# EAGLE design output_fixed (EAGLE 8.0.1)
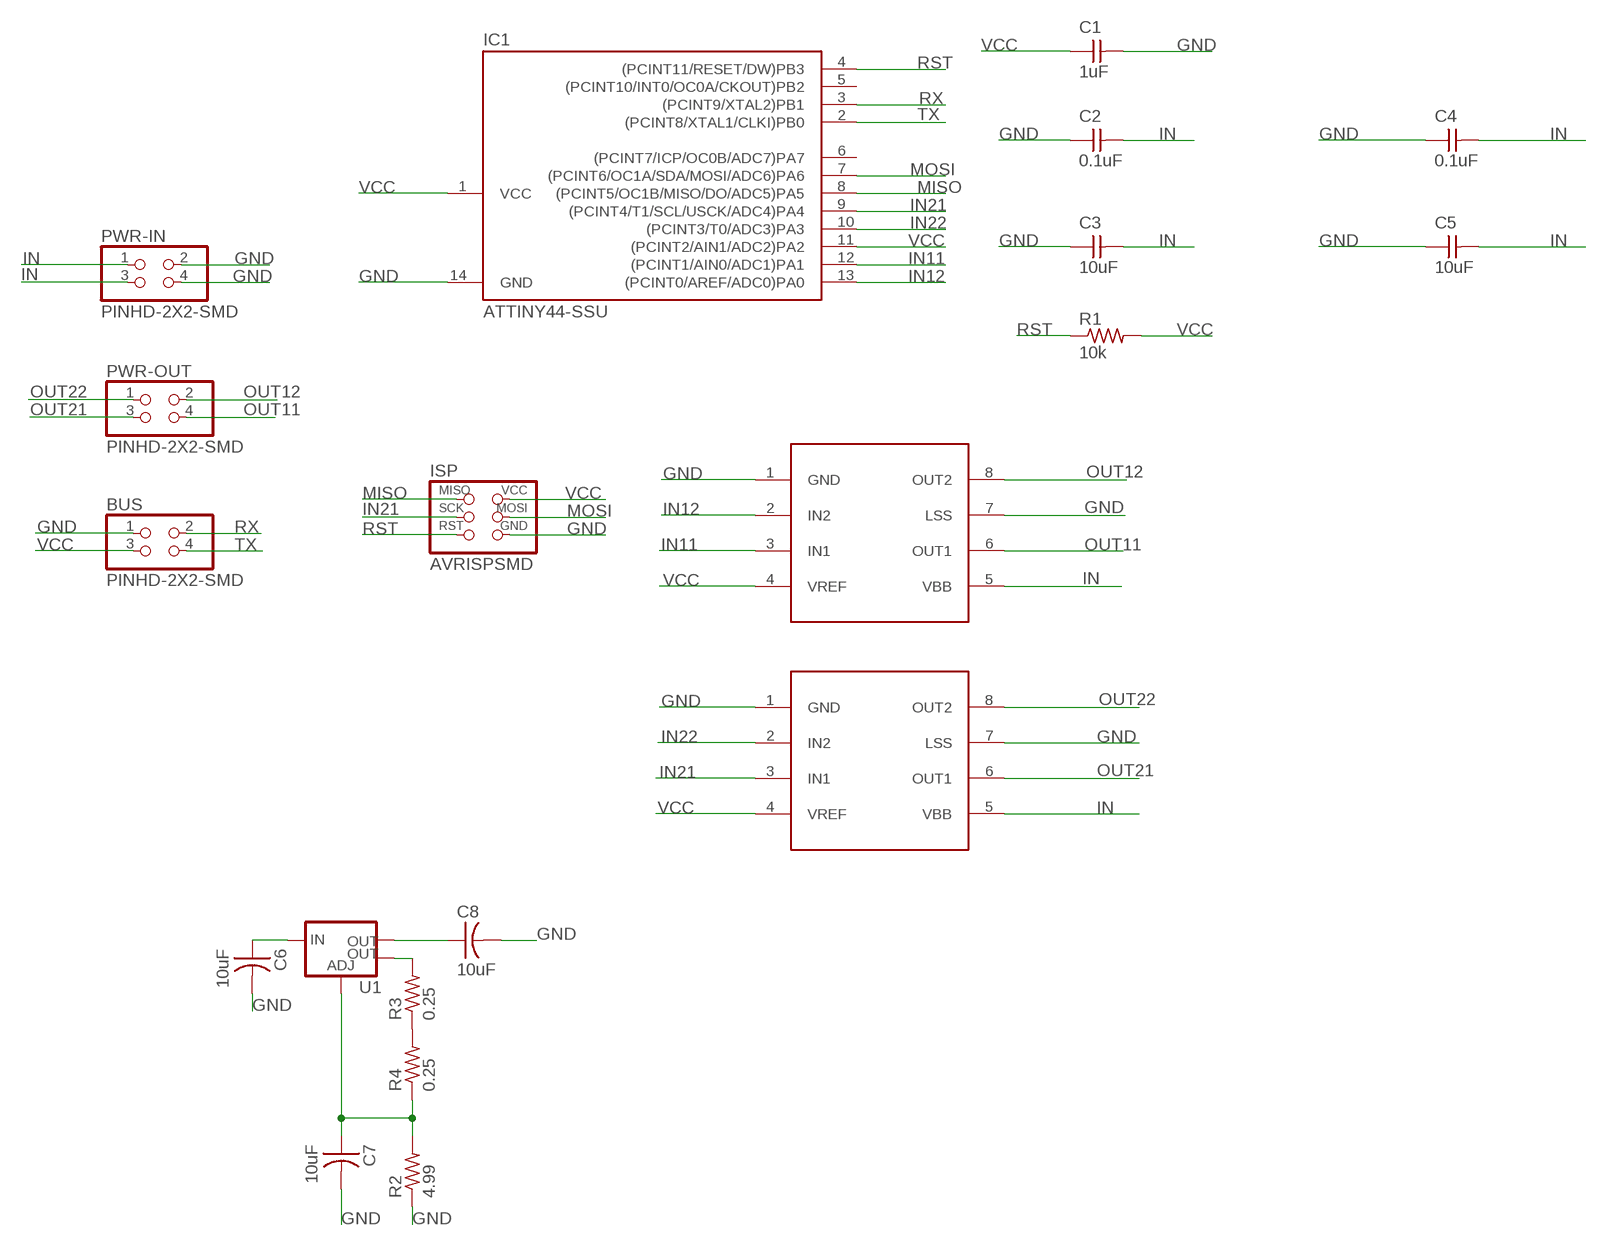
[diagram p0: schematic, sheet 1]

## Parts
BUS  PINHD-2X2-SMD  [2X02SMD]
C1  1uF  CAP-UNPOLARIZEDFAB  [C1206FAB]
C2  0.1uF  CAP-UNPOLARIZEDFAB  [C1206FAB]
C3  10uF  CAP-UNPOLARIZEDFAB  [C1206FAB]
C4  0.1uF  CAP-UNPOLARIZEDFAB  [C1206FAB]
C5  10uF  CAP-UNPOLARIZEDFAB  [C1206FAB]
C6  10uF  CAP-US1206FAB  [C1206FAB]
C7  10uF  CAP-US1206FAB  [C1206FAB]
C8  10uF  CAP-US1206FAB  [C1206FAB]
IC1  ATTINY44-SSU  [SOIC14]
ISP  AVRISPSMD  [2X03SMD]
PWR-IN  PINHD-2X2-SMD  [2X02SMD]
PWR-OUT  PINHD-2X2-SMD  [2X02SMD]
R1  10k  RES-US1206FAB  [R1206FAB]
R2  4.99  RES-US1206FAB  [R1206FAB]
R3  0.25  RES-US1206FAB  [R1206FAB]
R4  0.25  RES-US1206FAB  [R1206FAB]
U1  V_REG_LM1117SOT223  [SOT223]
U$5  A4953-H-BRIDGE-MOTOR-DRIVER  [SOIC8]
U$6  A4953-H-BRIDGE-MOTOR-DRIVER  [SOIC8]

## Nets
GND: BUS.1 C1.2 C2.1 C3.1 C4.1 C5.1 C6.2 C7.2 C8.2 IC1.14(GND) ISP.6(GND) PWR-IN.2 PWR-IN.4 R2.1 U$5.1(GND) U$5.7(LSS) U$6.1(GND) U$6.7(LSS)
IN: C2.2 C3.2 C4.2 C5.2 PWR-IN.1 PWR-IN.3 U$5.5(VBB) U$6.5(VBB)
IN11: IC1.12((PCINT1/AIN0/ADC1)PA1) U$5.3(IN1)
IN12: IC1.13((PCINT0/AREF/ADC0)PA0) U$5.2(IN2)
IN21: IC1.9((PCINT4/T1/SCL/USCK/ADC4)PA4) ISP.3(SCK) U$6.3(IN1)
IN22: IC1.10((PCINT3/T0/ADC3)PA3) U$6.2(IN2)
MISO: IC1.8((PCINT5/OC1B/MISO/DO/ADC5)PA5) ISP.1(MISO)
MOSI: IC1.7((PCINT6/OC1A/SDA/MOSI/ADC6)PA6) ISP.4(MOSI)
N$1: C6.1 U1.3(IN)
N$2: C7.1 R2.2 R4.1 U1.1(ADJ)
N$3: C8.1 U1.2(OUT)
N$4: R3.2 U1.4(OUT)
N$5: R3.1 R4.2
OUT11: PWR-OUT.4 U$5.6(OUT1)
OUT12: PWR-OUT.2 U$5.8(OUT2)
OUT21: PWR-OUT.3 U$6.6(OUT1)
OUT22: PWR-OUT.1 U$6.8(OUT2)
RST: IC1.4((PCINT11/RESET/DW)PB3) ISP.5(RST) R1.1
RX: BUS.2 IC1.3((PCINT9/XTAL2)PB1)
TX: BUS.4 IC1.2((PCINT8/XTAL1/CLKI)PB0)
VCC: BUS.3 C1.1 IC1.1(VCC) IC1.11((PCINT2/AIN1/ADC2)PA2) ISP.2(VCC) R1.2 U$5.4(VREF) U$6.4(VREF)
Unconnected: IC1.5((PCINT10/INT0/OC0A/CKOUT)PB2) IC1.6((PCINT7/ICP/OC0B/ADC7)PA7)

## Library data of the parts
BUS PWR-IN PWR-OUT = fab:PINHD-2X2-SMD
C1-C5 = fab:CAP-UNPOLARIZED
C6-C8 = fab:CAP-US
IC1 = fab:ATTINY44
ISP = fab:AVRISP
R1-R4 = fab:RES-US: Resistor (US Symbol)
U1 = fab:V_REG_LM1117: Voltage Regulator LM1117 Standard adjustable voltage regulator but in SMD form. Spark Fun Electronics SKU : COM-00595; PROD_ID: VREG-08170
U$5 U$6 = fab:A4953-H-BRIDGE-MOTOR-DRIVER

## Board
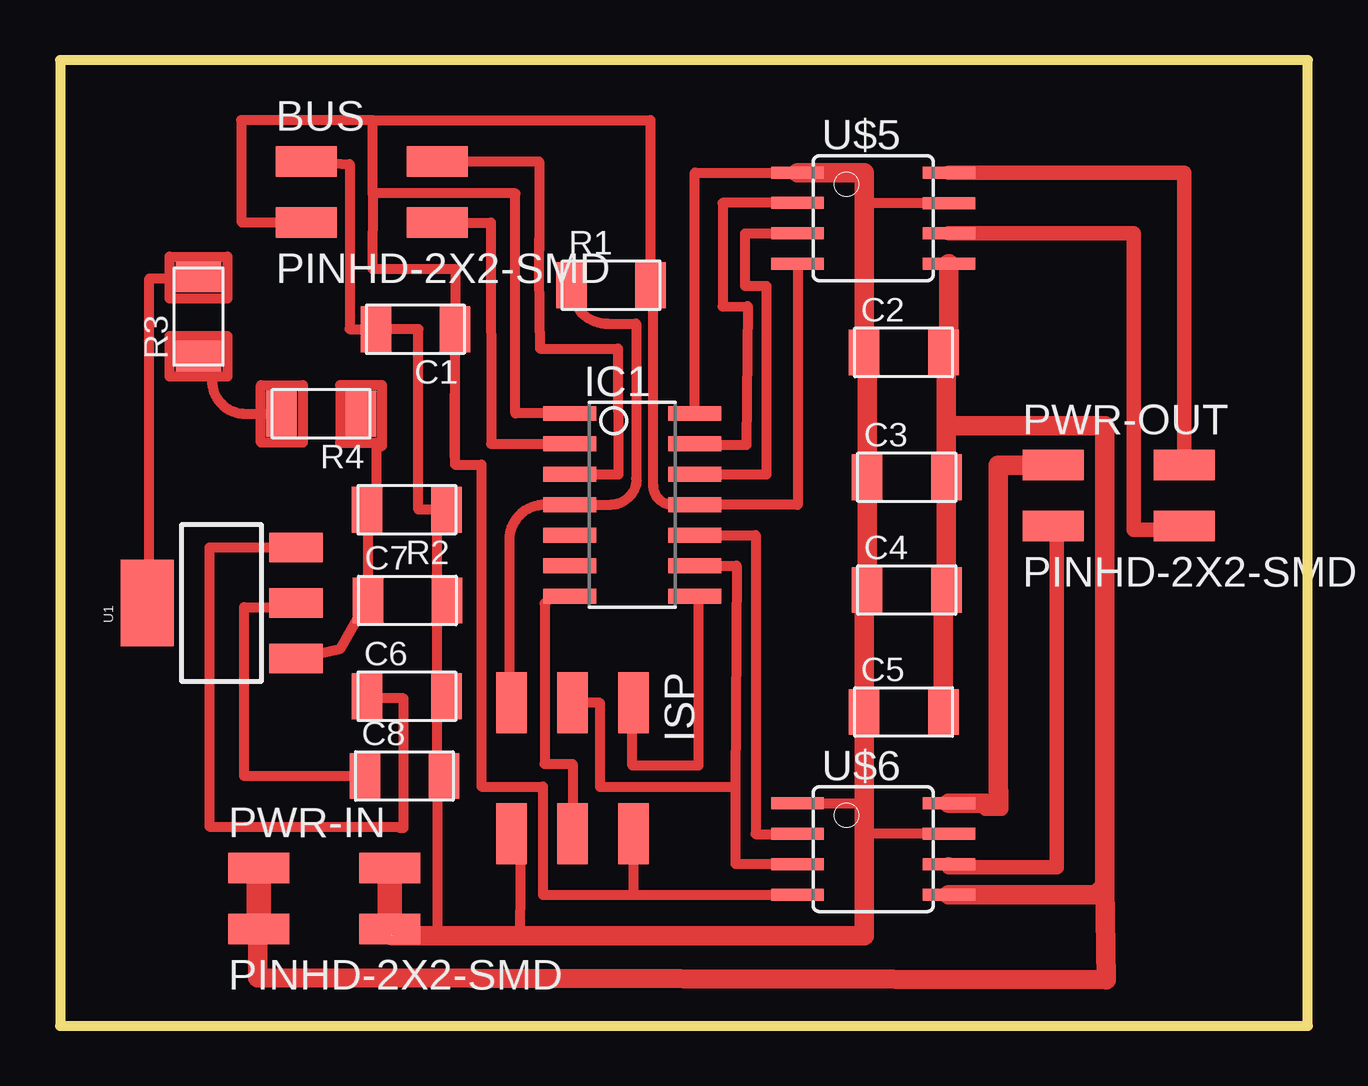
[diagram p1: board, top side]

Size 51.99 x 40.25 mm. Coordinates in mm from the lower left corner, seen from the top.
Outline: 0,0 51.99,0 51.99,40.25 0,40.25 0,0
Copper layers (1*16): Top 0.035mm / dielectric 1.5mm / Bottom 0.035mm
Design rules "default": minimum track width 10mil, minimum drill 24mil, track to track 8mil, track to pad 8mil, pad to pad 8mil, via to via 8mil, smd to smd 8mil, copper to edge 40mil, drill to drill 8mil, minimum pad ring 10mil, minimum via ring 8mil, stop-mask expansion 4mil, vias tented up to drill 0mil, thermal gap 10mil

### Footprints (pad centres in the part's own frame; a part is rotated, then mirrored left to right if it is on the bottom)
2X02SMD = smd 2.54 x 1.27: 1 -2.54,1.27; 2 2.92,1.27; 3 -2.54,-1.27; 4 2.92,-1.27
C1206FAB = smd 1.27 x 1.905: 1 -1.651,0; 2 1.651,0
SOIC14 = smd 0.61 x 2.21: 1 -3.81,-2.603; 2 -2.54,-2.603; 3 -1.27,-2.603; 4 0,-2.603; 5 1.27,-2.603; 6 2.54,-2.603; 7 3.81,-2.603; 8 3.81,2.603; 9 2.54,2.603; 10 1.27,2.603; 11 0,2.603; 12 -1.27,2.603; 13 -2.54,2.603; 14 -3.81,2.603
2X03SMD = smd 2.54 x 1.27: 1 -2.54,2.54; 2 2.92,2.54; 3 -2.54,0; 4 2.92,0; 5 -2.54,-2.54; 6 2.92,-2.54
R1206FAB = smd 1.27 x 1.905: 1 -1.651,0; 2 1.651,0
SOT223 = smd 1.219 x 2.235: 1 -2.311,-3.099; 2 0,-3.099; 3 2.311,-3.099 | smd 3.6 x 2.2: 4 0,3.099
SOIC8 = smd 0.5 x 2.2: 1 -1.905,-3.154; 2 -0.645,-3.154; 3 0.625,-3.154; 4 1.895,-3.154; 5 1.905,3.154; 6 0.635,3.154; 7 -0.635,3.154; 8 -1.905,3.154

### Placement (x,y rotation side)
BUS  12.8,34.75 0 top
C1  14.81,29.03 180 top
C2  35.15,28.07 0 top
C3  35.28,22.86 0 top
C4  35.28,18.16 0 top
C5  35.15,13.08 0 top
C6  14.45,13.74 0 top
C7  14.48,17.73 0 top
C8  14.35,10.41 0 top
IC1  23.85,21.72 270 top
ISP  21.36,10.92 270 top
PWR-IN  10.82,5.31 0 top
PWR-OUT  43.92,22.1 0 top
R1  22.96,30.86 0 top
R2  14.45,21.51 180 top
R3  5.77,29.56 90 top
R4  10.88,25.51 180 top
U1  6.73,17.62 90 top
U$5  33.88,33.66 270 top
U$6  33.88,7.37 270 top

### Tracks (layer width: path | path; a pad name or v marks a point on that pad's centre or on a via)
GND  (1 unrouted)
  Top 0.305: 15.72,21.51 R2.1 | C7.2 15.72,17.73 15.72,17.14 | C6.2 15.72,13.74 15.72,13.34 | C8.2 15.72,10.41 15.72,10.79
  Top 0.406: ISP.6 19.2,8.05 19.15,3.76 | U$6.7 33.5,8 | U$6.1 33.5,9.27 | U$5.7 33.5,34.29 | 33.5,25.53 33.63,25.65 | IC1.14 26.45,35.56 U$5.1 | BUS.1 12.06,35.92 12.06,29.03 C1.2 | C1.2 13.74,29.03 | C1.2 14.94,29.03 14.94,21.51 R2.1 | 15.72,21.51 15.72,17.14 15.72,13.34 15.72,10.79 15.72,3.76
  Top 0.813: 13.82,3.79 PWR-IN.2 | 13.84,3.76 15.72,3.76 19.15,3.76 33.5,3.76 33.5,8 33.5,9.27 C5.1 33.5,18.03 C4.1 C3.1 33.63,25.65 33.63,27.94 C2.1 33.5,34.29 33.5,35.56 U$5.1
  Top 1.016: PWR-IN.2 PWR-IN.4
IN
  Top 0.406: 36.8,18.16 C4.2 36.8,18.03 | C2.2 36.93,27.94 | PWR-IN.1 8.31,6.98 8.23,6.58
  Top 0.813: U$5.5 37.04,28.68 C2.2 | C5.2 36.8,18.03 | C4.2 C3.2 36.93,25.02 | 36.93,25.02 43.54,25.02 43.54,5.84 | 43.54,5.84 43.15,5.46 U$6.5 | 36.93,27.94 36.93,25.02 | 8.23,6.58 8.23,2.01 43.59,1.93 43.54,5.84
  Top 1.016: PWR-IN.1 PWR-IN.3
IN11
  Top 0.406: IC1.12 29.44,22.99 29.44,30.84 28.55,30.84 28.55,33.02 30.72,33.02 U$5.3
IN12
  Top 0.406: U$5.2 27.61,34.3 27.61,29.97 28.65,30 28.6,24.21 26.45,24.21 IC1.13
IN21
  Top 0.406: IC1.9 28.19,19.18 28.14,9.96 | 30.61,6.73 U$6.3 28.14,6.75 28.14,9.96 | 28.14,9.96 22.5,9.96 22.5,13.46 ISP.3
IN22
  Top 0.406: 30.59,8 U$6.2 30.73,8 28.98,8 28.98,20.45 IC1.10
MISO
  Top 0.406: IC1.8 26.59,17.91 26.59,10.85 23.85,10.85 23.85,13.46 ISP.1
MOSI
  Top 0.406: IC1.7 20.5,17.91 20.19,17.6 20.19,10.92 21.36,10.92 ISP.4 21.31,7.26
N$1
  Top 0.305: C6.1 12.8,13.55
  Top 0.406: U1.3 6.22,19.93 6.22,8.3 14.17,8.3 14.17,8.25 14.32,8.25 14.32,13.66 12.8,13.66 C6.1
N$2
  Top 0.305: 13.18,22.23 12.8,22.23 R2.2
  Top 0.406: 13.18,24.16 13.18,22.23 | U1.1 11.68,15.71 C7.1 12.83,21.51 R2.2 | 13.18,24.16 13.42,24.16 13.42,26.7 11.67,26.7 11.67,24.3 12.72,24.3 | 12.72,24.3 13.18,24.3 13.18,24.16 | 12.72,24.3 12.53,24.3 R4.1
N$3
  Top 0.305: 9.93,17.45 U1.2
  Top 0.406: C8.1 7.67,10.41 7.67,17.45 9.93,17.45
N$4
  Top 0.305: U1.4 3.72,17.27
  Top 0.406: 4.57,31.15 4.57,32.05 6.97,32.05 6.97,30.3 4.57,30.3 4.57,31.15 | 4.57,31.15 5.77,31.15 R3.2 | 4.57,31.15 3.72,31.15 3.72,17.27
N$5
  Top 0.305: R3.1 6.33,28.21
  Top 0.406: 6.33,28.21 6.33,27.05 | 6.33,27.05 4.57,27.05 4.57,28.76 6.97,28.76 6.97,27.05 6.33,27.05 | 6.33,27.05 6.33,26.89 arc90 7.72,25.5 8.37,25.5 | 8.37,25.5 R4.2 | R4.2 arc90 R4.2 | 8.37,25.5 8.37,26.7 10.12,26.7 10.12,24.3 8.37,24.3 8.37,25.5
OUT11
  Top 0.406: 46.84,20.68 PWR-OUT.4
  Top 0.61: U$5.6 44.73,33.02 44.73,20.68 46.84,20.68
OUT12
  Top 0.61: U$5.8 46.84,35.56 PWR-OUT.2
OUT21
  Top 0.61: PWR-OUT.3 41.53,20.83 41.53,6.6 37.04,6.6 U$6.6
OUT22
  Top 0.61: 39.09,9.78 39.22,9.78 39.22,9.04 38.58,9.04 38.58,9.27
  Top 0.813: U$6.8 38.58,9.27 | 39.09,9.78 39.09,23.37 PWR-OUT.1
RST
  Top 0.406: 21.25,21.67 IC1.4 | IC1.4 20.18,21.72 arc90 18.72,20.25 18.72,13.46 ISP.5 | IC1.4 22.93,21.72 arc90 24.02,22.8 24,22.8 24,29.26 22.82,29.26 22.82,29.26 arc-90 21.31,30.77 R1.1
RX
  Top 0.406: IC1.3 23.27,22.99 23.24,28.12 23.24,28.22 19.99,28.22 19.99,28.91 19.97,32.31 | 19.97,32.31 19.96,32.79 | BUS.2 19.97,36.02 19.97,32.31
TX
  Top 0.406: BUS.4 17.96,33.48 17.96,24.26 IC1.2
VCC
  Top 0.406: U$5.4 30.73,21.72 IC1.11 25.51,21.72 arc-90 24.72,22.5 24.72,30.86 R1.2 | 23.77,7.37 ISP.2 | 16.45,23.7 16.45,23.39 17.56,23.39 17.56,9.97 20.12,9.97 20.12,5.46 23.88,5.46 | 16.45,23.7 C1.1 | R1.2 24.61,37.74 13.03,37.74 | 13.03,37.74 7.57,37.74 | 24.74,30.73 R1.2 | 21.25,25.48 IC1.1 18.98,25.53 18.98,34.7 13.06,34.7 | ISP.2 23.88,8 23.8,7.62 | C1.1 16.46,31.55 13.03,31.55 13.06,34.7 | 13.06,34.7 13.03,34.7 13.03,37.74 | 7.54,37.74 7.57,37.74 | 7.57,37.74 7.57,33.48 BUS.3 | C1.1 16.45,23.7 | 23.88,5.46 23.93,5.56 | U$6.4 30.68,5.46 23.88,5.46 | ISP.2 23.88,8 23.88,5.46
